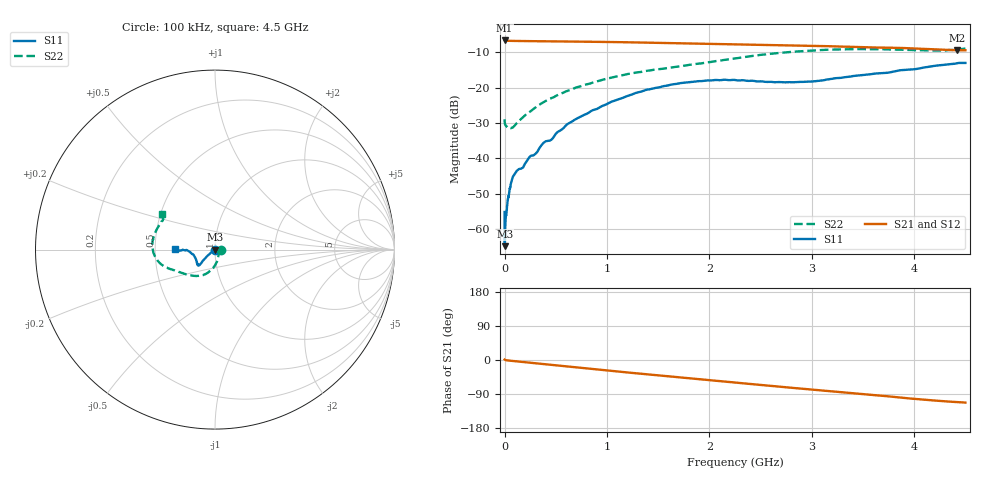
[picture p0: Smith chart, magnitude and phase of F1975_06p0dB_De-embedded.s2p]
! Integrated Device Technology
! Corporate Headquarters
! 6024 Silver Creek Valley Road
! San Jose, CA 95138  USA
! Phone:  1-408-284-8200
! Toll Free:  1-800-223-1366
! Webpage:  http://www.idt.com/
! Timing and RF Division
! 515 Groton Road, Suite 102
! Westford, MA 01886-6024
! Device:  F1975
! Description: 6-bit, 75 ohm, 0.5 dB Digital Step Attenuator
! Frequency:  5.0 MHz -  3.00 GHz
! Package:  4x4 mm QFN Plastic Package: 20 pin
! Ports:  2 RF, 11 DC
!  Pin  1  = D5 (16 dB)
!  Pin  2  = RF1  =  Port 1
!  Pin  3  = Serial Data In (DATA)
!  Pin  4  = Serial Clock (CLK)
!  Pin  5  = Serial Latch Enable (LE)
!  Pin  6  = VDD
!  Pin  7  = NC
!  Pin  8  = NC
!  Pin  9  = NC
!  Pin 10  = GND
!  Pin 11  = GND
!  Pin 12  = NC
!  Pin 13  = VMODE
!  Pin 14  = RF2  =  Port 2
!  Pin 15  = D4 (8 dB)
!  Pin 16  = D3 (4 dB)
!  Pin 17  = D2 (2 dB)
!  Pin 18  = NC
!  Pin 19  = D1 (1 dB)
!  Pin 20  = D0 (0.5 dB)
! State:  12
! Atten State:  6.0 dB
! Voltage:  +3.30 Volts
! Current:  0.595 mA
! Data:  The device was measured on a F1975 evaluation board which has
!  individual transmission lines to the RF pins.  Data was collected
!  using a calibrated network analyzer.  The evaluation board was
!  de-embedded using Automatic Fixture Removal (AFR).
!  The reference plane is the edge of the package pin.
! Misc:
!  Action Tracker AT0415
! Date Measured:  2018-02-08
! Date:  2018-03-26  MJV
! Note:
!  Integrated Device Technology supplies this data as a sample of measured
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# GHz S dB R 75
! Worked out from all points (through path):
!   291 points, 100 kHz to 4.5 GHz, reference 75 ohm
!   highest |S21| = -6.67 dB at 100 kHz (marker M1); lowest = -9.4 dB at 4.42 GHz (marker M2)
!   group delay of S21, straight-line fit = 70.9 ps
!   lowest |S11| = -64.8 dB at 2 MHz (marker M3), VSWR 1.00, Z = 75 - j0.0844 ohm
!   |S11| at or under -10 dB: start of sweep to end of sweep
!   |S22| runs from -31.5 to -8.9 dB; largest |S21 - S12| = 0.00022
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0.0001  -55.14 -2.2  -6.67 1.2  -6.67 1.2  -28.93 -0.2
0.0004  -60.66 -27.9  -6.69 1.1  -6.69 1.1  -29.40 -2.2
0.0005  -60.10 -37.3  -6.69 1.1  -6.69 1.1  -29.53 -2.2
0.0006  -61.34 -31.8  -6.69 1.1  -6.69 1.1  -29.64 -2.6
0.0007  -60.36 -31.8  -6.70 1.0  -6.70 1.0  -29.71 -2.7
0.0008  -61.67 -51.7  -6.70 1.0  -6.70 1.0  -29.76 -2.6
0.0009  -60.90 -48.1  -6.70 1.0  -6.70 1.0  -29.84 -2.4
0.002  -64.80 -77.9  -6.71 0.8  -6.71 0.8  -30.11 -2.8
0.005  -60.27 -105.5  -6.72 0.3  -6.72 0.3  -30.34 -5.0
0.008  -58.27 -107.9  -6.73 -0.2  -6.73 -0.2  -30.56 -7.5
0.023  -53.45 -132.9  -6.75 -0.9  -6.75 -0.9  -31.09 -14.4
0.05  -48.49 -138.6  -6.78 -1.7  -6.78 -1.7  -31.36 -24.6
0.08  -45.22 -132.2  -6.80 -2.6  -6.80 -2.6  -31.25 -37.0
0.38  -35.61 -136.9  -6.90 -10.8  -6.90 -10.8  -24.12 -78.2
0.76  -27.93 -140.9  -7.01 -21.0  -7.01 -21.0  -19.43 -97.4
1.04  -24.03 -139.8  -7.11 -28.6  -7.11 -28.6  -17.17 -108.5
1.52  -19.85 -136.0  -7.34 -41.2  -7.34 -41.2  -14.74 -126.9
2.26  -17.88 -139.5  -7.76 -59.8  -7.75 -59.8  -11.70 -154.0
3.02  -18.22 -166.1  -8.21 -78.6  -8.20 -78.6  -9.49 -173.2
3.76  -15.70 -178.6  -8.71 -96.2  -8.71 -96.2  -9.21 164.2
4.42  -13.09 -178.9  -9.44 -111.0  -9.44 -111.0  -9.16 147.4
4.5  -13.02 179.0  -9.42 -112.4  -9.42 -112.4  -8.93 146.0
